(* Logix 5000 Routine export GOV_Plus_Program; software revision 20.01 *)

TYPE GOVPlus_Output :
STRUCT
   Target : DINT;
   Actuator_Control : INT;
   StatusControl : INT;
   Stop : BOOL;
   Reserved18 : BOOL;
   Reserved19 : BOOL;
   Reserved20 : BOOL;
   Reserved21 : BOOL;
   Reserved22 : BOOL;
   Reserved23 : BOOL;
   Reserved24 : BOOL;
   Reserved25 : BOOL;
   Reserved26 : BOOL;
   Reserved27 : BOOL;
   Reserved28 : BOOL;
   Reserved29 : BOOL;
   SW1_Failsafe : BOOL;
   SW1_Latching : BOOL;
   SW1_Enabled : BOOL;
   Spare : INT;
   Aux_Out : REAL;
   Float_Val : DINT;
   Float_Div : DINT;
END_STRUCT
END_TYPE

TYPE GOVPlus_ProgramData :
STRUCT
   GOV_ComCode : INT;
   GOV_ComCount : INT;
   GOV_Reconfigure : BOOL;
   Refresh_Stop_Data : BOOL;
   Refresh_ONS : BOOL;
   Stop_ONS : BOOL;
   Stop_Out_at_Stop : BOOL;
   Safety_Loop_at_Stop : BOOL;
   Actuator_Mode_Backup : BOOL;
   Current_Limit_Backup : BOOL;
   Reconfigure_Req : BOOL;
   Reconfigure_ONS : BOOL;
   Load_Defaults : BOOL;
   Limit_Low : REAL;
   Limit_High : REAL;
   Aux_Limit_Low : REAL;
   Aux_Limit_High : REAL;
   Stop_Data : GOV_Stop_Data;
   Gearteeth_Backup : INT;
   Start_Speed_Backup : DINT;
   Crank_Speed_Backup : DINT;
   Overspeed_Backup : DINT;
   Output_at_0_Percent_Backup : REAL;
   Output_at_100_Percent_Backup : REAL;
END_STRUCT
END_TYPE

TYPE GOVPlus_Input :
STRUCT
   Reserved1 : BOOL;
   Reserved2 : BOOL;
   V3_3Low : BOOL;
   V3_3High : BOOL;
   V5Low : BOOL;
   V5High : BOOL;
   V12_5Low : BOOL;
   V12_5High : BOOL;
   V24Low : BOOL;
   V24High : BOOL;
   AuxLoopLow : BOOL;
   AuxLoopHigh : BOOL;
   Reserved13 : BOOL;
   Reserved14 : BOOL;
   DemandLoopLow : BOOL;
   DemandLoopHigh : BOOL;
   CoolDownInputStatus : BOOL;
   StopInputStatus : BOOL;
   CurrentLoopOutputOpen : BOOL;
   SW1_Enabled_Echo : BOOL;
   SW1_Latching_Echo : BOOL;
   SW1_Failsafe_Echo : BOOL;
   Reserved23 : BOOL;
   Rotating : BOOL;
   AlarmOutActive : BOOL;
   StopOutClosed : BOOL;
   AuxOutputOutOfRange : BOOL;
   Target_Met : BOOL;
   Stop_Echo : BOOL;
   Reserved30 : BOOL;
   VoltOutActive : BOOL;
   V12_5SupplyFaulted : BOOL;
   Breaking : BOOL;
   WatchdogFailure : BOOL;
   FactoryCalEnabled : BOOL;
   WatchdogInhibited : BOOL;
   ActuatorEnabled : BOOL;
   Governing : BOOL;
   Timer1Active : BOOL;
   Timer2Active : BOOL;
   Timer3Active : BOOL;
   Purging : BOOL;
   Cooldown : BOOL;
   Max_Authority : BOOL;
   Demand_Active : BOOL;
   Target_Active : BOOL;
   Voltage_Driver_Output_On : BOOL;
   Reserved48 : BOOL;
   Aux_Output_Alarm : BOOL;
   Actuator_Output_Fault : BOOL;
   Overspeed : BOOL;
   Underspeed : BOOL;
   Stopped : BOOL;
   Reserved54 : BOOL;
   Reserved55 : BOOL;
   Reserved56 : BOOL;
   Reserved57 : BOOL;
   Reserved58 : BOOL;
   Reserved59 : BOOL;
   Reserved60 : BOOL;
   Reserved61 : BOOL;
   Reserved62 : BOOL;
   Reserved63 : BOOL;
   Reserved64 : BOOL;
   GovTime : REAL;
   Accelleration : REAL;
   RPM : DINT;
   RPMUnfiltered : REAL;
   DemandInput : REAL;
   AuxInput : REAL;
   CurrentOut : REAL;
   VoltageOut : REAL;
   Voltage_240 : REAL;
   Voltage_100 : REAL;
   Voltage_50 : REAL;
   Voltage_33 : REAL;
   Voltage_Output_Sense_Value : REAL;
   DemandTarget : DINT;
   ProcessorUsage : INT;
   GovState : INT;
   Speed_Target : REAL;
   Acceleration_Target : REAL;
   Acceleration_Error : REAL;
   RPM_Error : INT;
   Actuator_Position_Output : INT;
   ActuatorCounts : DINT;
   UpWindow : INT;
   DownWindow : INT;
   Float_Rsp : REAL;
   Comm_Status : INT;
   Spare_Echo : INT;
   Aux_Out_Echo : REAL;
END_STRUCT
END_TYPE

TYPE GOV_Stop_Data :
STRUCT
   Warmup_1 : BOOL;
   Warmup_2 : BOOL;
   Warmup_3 : BOOL;
   Cooldown : BOOL;
   Demand : BOOL;
   Purging : BOOL;
   Actuator_Offline : BOOL;
   Governing : BOOL;
   Braking : BOOL;
   Max_Authority : BOOL;
   Target_Met : BOOL;
   Underspeed : BOOL;
   Alarm : BOOL;
   V24Problem : BOOL;
   V12Problem : BOOL;
   PowerProblem : BOOL;
   Actuator_Output : INT;
   Target : DINT;
   RPM : DINT;
   Acceleration : INT;
   RPM_Error : INT;
   Acceleration_Target : INT;
   Acceleration_Error : INT;
   Actuator_Position : INT;
   Reserved : INT;
END_STRUCT
END_TYPE

VAR_GLOBAL   (* controller tags *)
   GOV_Input : GOVPlus_Input := (SW1_Enabled_Echo := 1, SW1_Latching_Echo := 1, SW1_Failsafe_Echo := 1, AlarmOutActive := 1, StopOutClosed := 1, Stop_Echo := 1, VoltOutActive := 1, WatchdogFailure := 1, Demand_Active := 1, Target_Active := 1, Underspeed := 1, DemandInput := 18.0, AuxInput := 4.959961, CurrentOut := 4.0, VoltageOut := 9.98999, Voltage_240 := 22.899902, Voltage_100 := 12.399902, Voltage_50 := 5.2999268, Voltage_33 := 3.1999512, Voltage_Output_Sense_Value := 9.899902, DemandTarget := 1801, ProcessorUsage := 34, UpWindow := 5, DownWindow := 5, Float_Rsp := 2.3999634, Aux_Out_Echo := 10.0);
   GOV_Stop_MSG : MESSAGE;
        MessageParameters(MessageType := CIP Generic, ConnectedFlag := 2, ConnectionPath := GOVPlus, ServiceCode := 16#0001, ObjectType := 16#006e, TargetObject := 1, DestinationTag := GOV_Program_Data.Stop_Data)
   GOVPlus_NFO : MESSAGE;
        MessageParameters(MessageType := Module Reconfigure, RequestedLength := 1, ConnectionPath := GOVPlus)
   GOV_Output : GOVPlus_Output := (Target := 1800, Actuator_Control := 15, Stop := 1, SW1_Failsafe := 1, SW1_Latching := 1, SW1_Enabled := 1, Aux_Out := 10.0, Float_Val := 240, Float_Div := 100);
   GOV_Program_Data : GOVPlus_ProgramData := (Actuator_Mode_Backup := 1, Limit_Low := 4.0, Limit_High := 20.0, Aux_Limit_High := 10.0, Stop_Data.Underspeed := 1, Stop_Data.Alarm := 1, Gearteeth_Backup := 60, Start_Speed_Backup := 150, Crank_Speed_Backup := 50, Overspeed_Backup := 2000, Output_at_0_Percent_Backup := 4.0, Output_at_100_Percent_Backup := 20.0);
END_VAR

PROGRAM DET_COM

ROUTINE GOV_Plus_Program   (* ladder *)
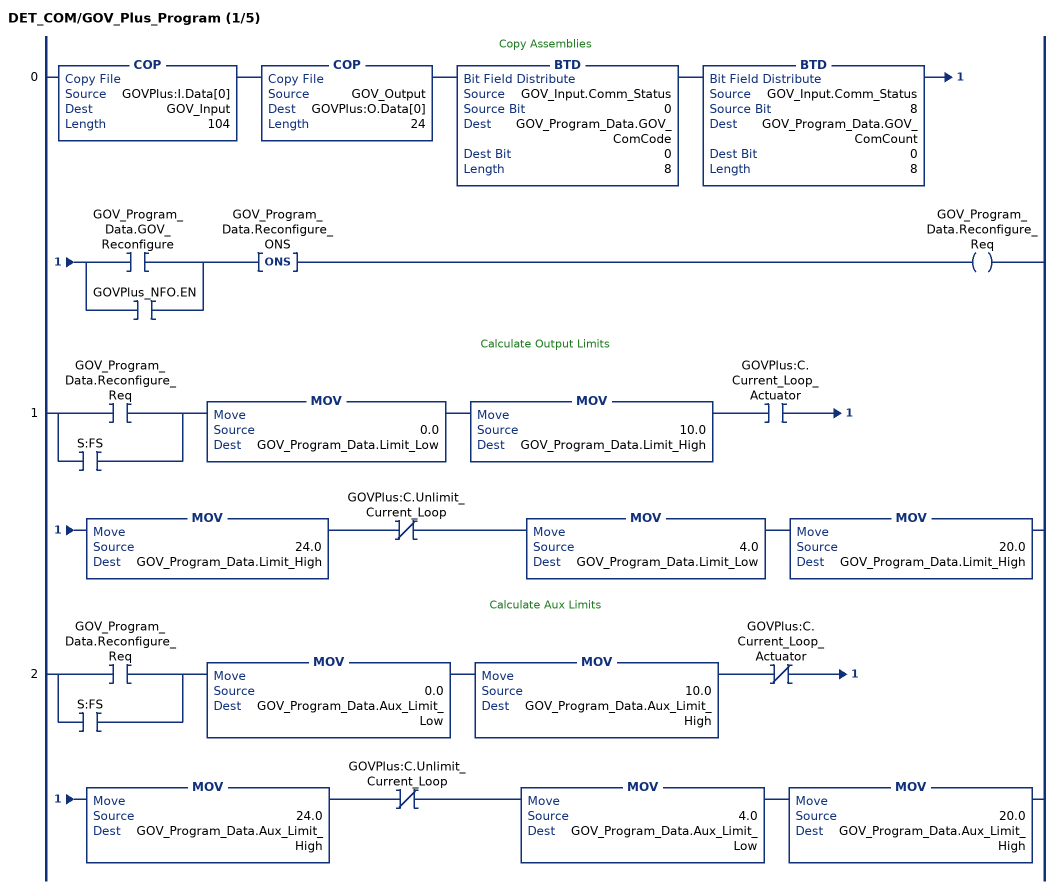
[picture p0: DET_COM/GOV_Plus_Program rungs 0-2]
   // Copy Assemblies
   0: COP(GOVPlus:I.Data[0],GOV_Input,104)COP(GOV_Output,GOVPlus:O.Data[0],24)BTD(GOV_Input.Comm_Status,0,GOV_Program_Data.GOV_ComCode,0,8)BTD(GOV_Input.Comm_Status,8,GOV_Program_Data.GOV_ComCount,0,8)[XIC(GOV_Program_Data.GOV_Reconfigure) ,XIC(GOVPlus_NFO.EN) ]ONS(GOV_Program_Data.Reconfigure_ONS)OTE(GOV_Program_Data.Reconfigure_Req);
   // Calculate Output Limits
   1: [XIC(GOV_Program_Data.Reconfigure_Req) ,XIC(S:FS) ]MOV(0.0,GOV_Program_Data.Limit_Low)MOV(10.0,GOV_Program_Data.Limit_High)XIC(GOVPlus:C.Current_Loop_Actuator)MOV(24.0,GOV_Program_Data.Limit_High)XIO(GOVPlus:C.Unlimit_Current_Loop)MOV(4.0,GOV_Program_Data.Limit_Low)MOV(20.0,GOV_Program_Data.Limit_High);
   // Calculate Aux Limits
   2: [XIC(GOV_Program_Data.Reconfigure_Req) ,XIC(S:FS) ]MOV(0.0,GOV_Program_Data.Aux_Limit_Low)MOV(10.0,GOV_Program_Data.Aux_Limit_High)XIO(GOVPlus:C.Current_Loop_Actuator)MOV(24.0,GOV_Program_Data.Aux_Limit_High)XIO(GOVPlus:C.Unlimit_Current_Loop)MOV(4.0,GOV_Program_Data.Aux_Limit_Low)MOV(20.0,GOV_Program_Data.Aux_Limit_High);
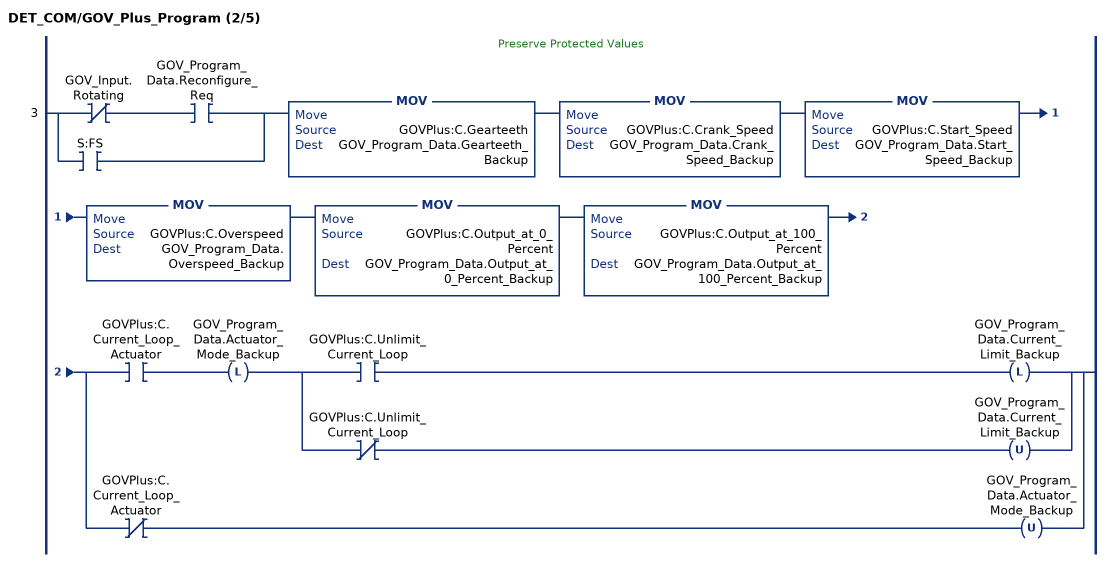
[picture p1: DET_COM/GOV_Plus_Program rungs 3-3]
   // Preserve Protected Values
   3: [XIO(GOV_Input.Rotating) XIC(GOV_Program_Data.Reconfigure_Req) ,XIC(S:FS) ]MOV(GOVPlus:C.Gearteeth,GOV_Program_Data.Gearteeth_Backup)MOV(GOVPlus:C.Crank_Speed,GOV_Program_Data.Crank_Speed_Backup)MOV(GOVPlus:C.Start_Speed,GOV_Program_Data.Start_Speed_Backup)MOV(GOVPlus:C.Overspeed,GOV_Program_Data.Overspeed_Backup)MOV(GOVPlus:C.Output_at_0_Percent,GOV_Program_Data.Output_at_0_Percent_Backup)MOV(GOVPlus:C.Output_at_100_Percent,GOV_Program_Data.Output_at_100_Percent_Backup)[XIC(GOVPlus:C.Current_Loop_Actuator) OTL(GOV_Program_Data.Actuator_Mode_Backup) [XIC(GOVPlus:C.Unlimit_Current_Loop) OTL(GOV_Program_Data.Current_Limit_Backup) ,XIO(GOVPlus:C.Unlimit_Current_Loop) OTU(GOV_Program_Data.Current_Limit_Backup) ] ,XIO(GOVPlus:C.Current_Loop_Actuator) OTU(GOV_Program_Data.Actuator_Mode_Backup) ];
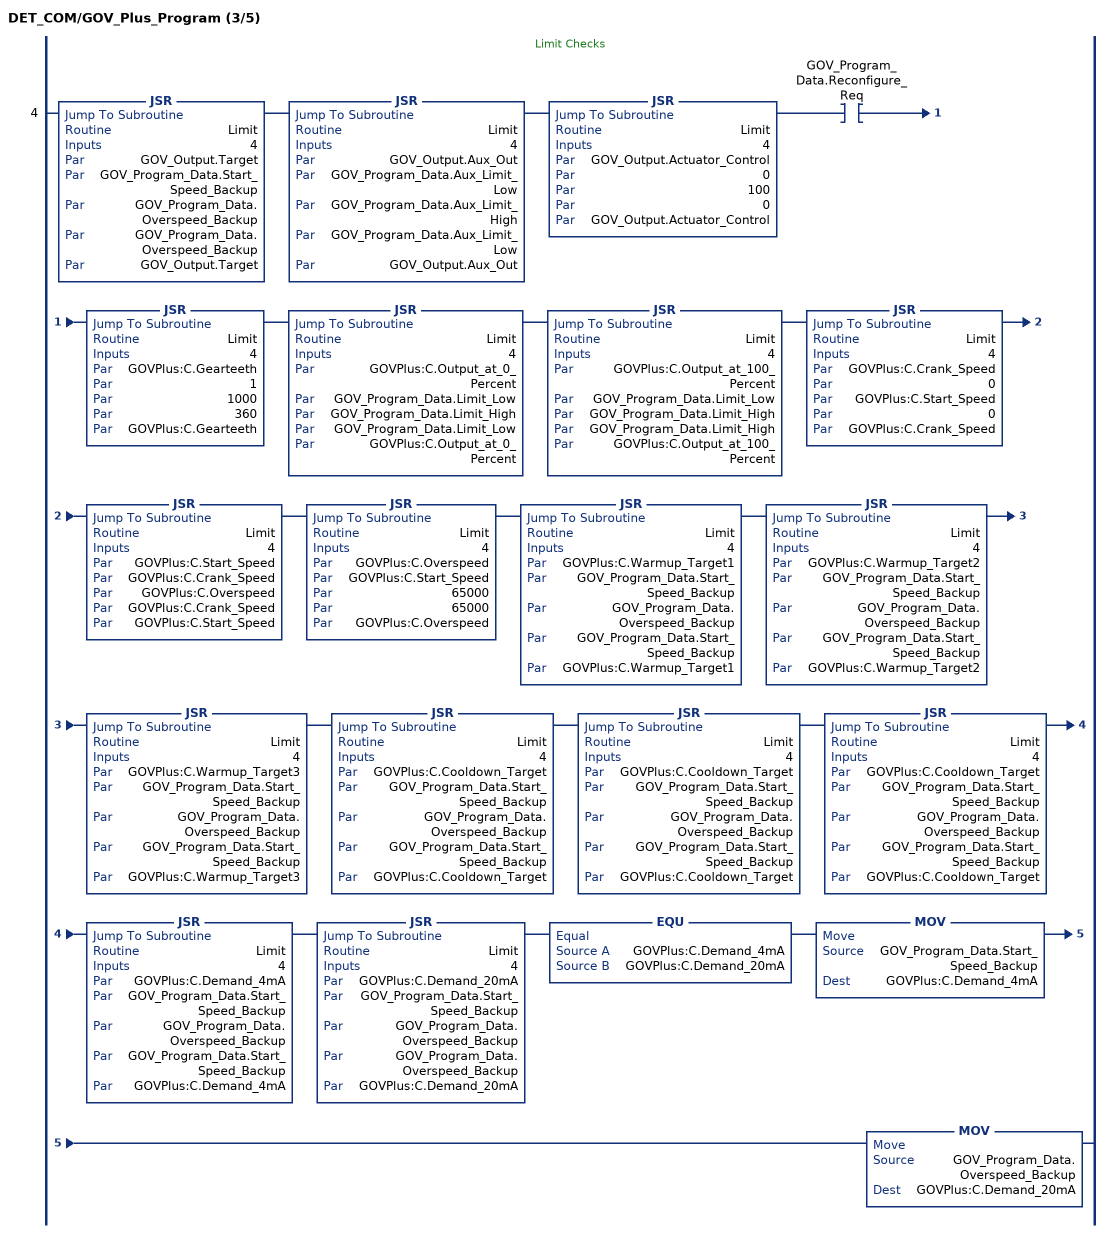
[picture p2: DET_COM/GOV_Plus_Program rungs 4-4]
   // Limit Checks
   4: JSR(Limit,4,GOV_Output.Target,GOV_Program_Data.Start_Speed_Backup,GOV_Program_Data.Overspeed_Backup,GOV_Program_Data.Overspeed_Backup,GOV_Output.Target)JSR(Limit,4,GOV_Output.Aux_Out,GOV_Program_Data.Aux_Limit_Low,GOV_Program_Data.Aux_Limit_High,GOV_Program_Data.Aux_Limit_Low,GOV_Output.Aux_Out)JSR(Limit,4,GOV_Output.Actuator_Control,0,100,0,GOV_Output.Actuator_Control)XIC(GOV_Program_Data.Reconfigure_Req)JSR(Limit,4,GOVPlus:C.Gearteeth,1,1000,360,GOVPlus:C.Gearteeth)JSR(Limit,4,GOVPlus:C.Output_at_0_Percent,GOV_Program_Data.Limit_Low,GOV_Program_Data.Limit_High,GOV_Program_Data.Limit_Low,GOVPlus:C.Output_at_0_Percent)JSR(Limit,4,GOVPlus:C.Output_at_100_Percent,GOV_Program_Data.Limit_Low,GOV_Program_Data.Limit_High,GOV_Program_Data.Limit_High,GOVPlus:C.Output_at_100_Percent)JSR(Limit,4,GOVPlus:C.Crank_Speed,0,GOVPlus:C.Start_Speed,0,GOVPlus:C.Crank_Speed)JSR(Limit,4,GOVPlus:C.Start_Speed,GOVPlus:C.Crank_Speed,GOVPlus:C.Overspeed,GOVPlus:C.Crank_Speed,GOVPlus:C.Start_Speed)JSR(Limit,4,GOVPlus:C.Overspeed,GOVPlus:C.Start_Speed,65000,65000,GOVPlus:C.Overspeed)JSR(Limit,4,GOVPlus:C.Warmup_Target1,GOV_Program_Data.Start_Speed_Backup,GOV_Program_Data.Overspeed_Backup,GOV_Program_Data.Start_Speed_Backup,GOVPlus:C.Warmup_Target1)JSR(Limit,4,GOVPlus:C.Warmup_Target2,GOV_Program_Data.Start_Speed_Backup,GOV_Program_Data.Overspeed_Backup,GOV_Program_Data.Start_Speed_Backup,GOVPlus:C.Warmup_Target2)JSR(Limit,4,GOVPlus:C.Warmup_Target3,GOV_Program_Data.Start_Speed_Backup,GOV_Program_Data.Overspeed_Backup,GOV_Program_Data.Start_Speed_Backup,GOVPlus:C.Warmup_Target3)JSR(Limit,4,GOVPlus:C.Cooldown_Target,GOV_Program_Data.Start_Speed_Backup,GOV_Program_Data.Overspeed_Backup,GOV_Program_Data.Start_Speed_Backup,GOVPlus:C.Cooldown_Target)JSR(Limit,4,GOVPlus:C.Cooldown_Target,GOV_Program_Data.Start_Speed_Backup,GOV_Program_Data.Overspeed_Backup,GOV_Program_Data.Start_Speed_Backup,GOVPlus:C.Cooldown_Target)JSR(Limit,4,GOVPlus:C.Cooldown_Target,GOV_Program_Data.Start_Speed_Backup,GOV_Program_Data.Overspeed_Backup,GOV_Program_Data.Start_Speed_Backup,GOVPlus:C.Cooldown_Target)JSR(Limit,4,GOVPlus:C.Demand_4mA,GOV_Program_Data.Start_Speed_Backup,GOV_Program_Data.Overspeed_Backup,GOV_Program_Data.Start_Speed_Backup,GOVPlus:C.Demand_4mA)JSR(Limit,4,GOVPlus:C.Demand_20mA,GOV_Program_Data.Start_Speed_Backup,GOV_Program_Data.Overspeed_Backup,GOV_Program_Data.Overspeed_Backup,GOVPlus:C.Demand_20mA)EQU(GOVPlus:C.Demand_4mA,GOVPlus:C.Demand_20mA)MOV(GOV_Program_Data.Start_Speed_Backup,GOVPlus:C.Demand_4mA)MOV(GOV_Program_Data.Overspeed_Backup,GOVPlus:C.Demand_20mA);
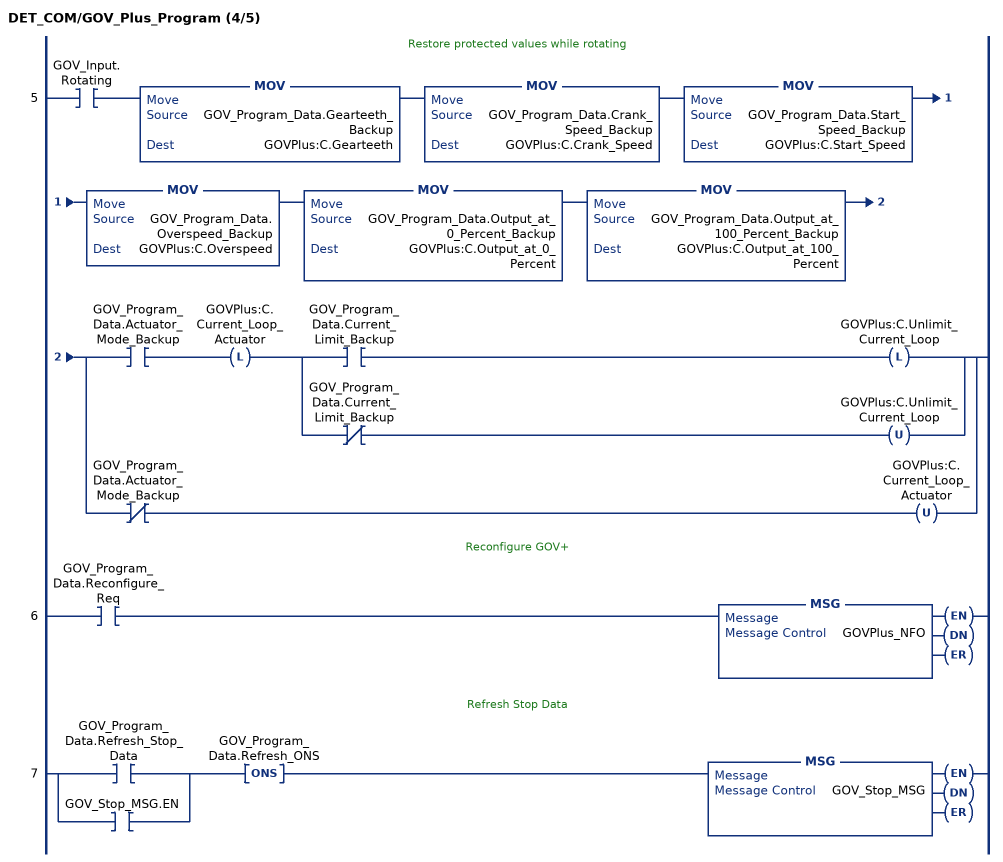
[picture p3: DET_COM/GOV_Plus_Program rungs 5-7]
   // Restore protected values while rotating
   5: XIC(GOV_Input.Rotating)MOV(GOV_Program_Data.Gearteeth_Backup,GOVPlus:C.Gearteeth)MOV(GOV_Program_Data.Crank_Speed_Backup,GOVPlus:C.Crank_Speed)MOV(GOV_Program_Data.Start_Speed_Backup,GOVPlus:C.Start_Speed)MOV(GOV_Program_Data.Overspeed_Backup,GOVPlus:C.Overspeed)MOV(GOV_Program_Data.Output_at_0_Percent_Backup,GOVPlus:C.Output_at_0_Percent)MOV(GOV_Program_Data.Output_at_100_Percent_Backup,GOVPlus:C.Output_at_100_Percent)[XIC(GOV_Program_Data.Actuator_Mode_Backup) OTL(GOVPlus:C.Current_Loop_Actuator) [XIC(GOV_Program_Data.Current_Limit_Backup) OTL(GOVPlus:C.Unlimit_Current_Loop) ,XIO(GOV_Program_Data.Current_Limit_Backup) OTU(GOVPlus:C.Unlimit_Current_Loop) ] ,XIO(GOV_Program_Data.Actuator_Mode_Backup) OTU(GOVPlus:C.Current_Loop_Actuator) ];
   // Reconfigure GOV+
   6: XIC(GOV_Program_Data.Reconfigure_Req)MSG(GOVPlus_NFO);
   // Refresh Stop Data
   7: [XIC(GOV_Program_Data.Refresh_Stop_Data) ,XIC(GOV_Stop_MSG.EN) ]ONS(GOV_Program_Data.Refresh_ONS)MSG(GOV_Stop_MSG);
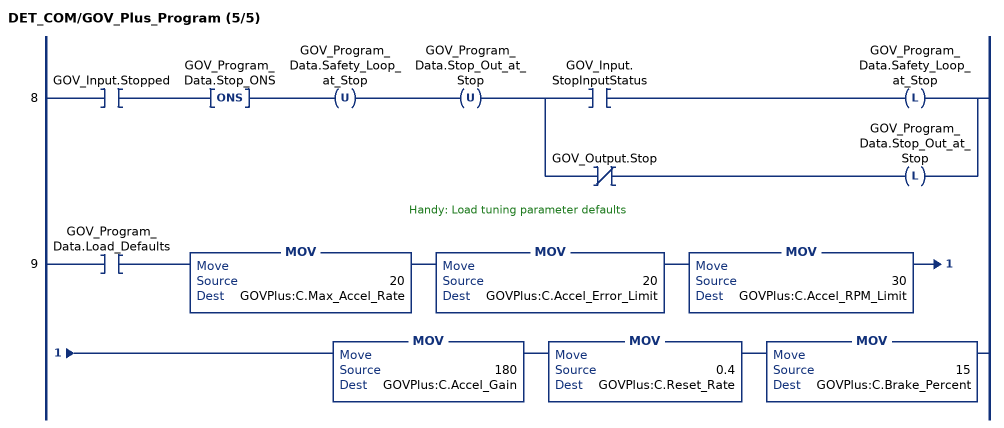
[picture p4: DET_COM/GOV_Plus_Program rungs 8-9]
   8: XIC(GOV_Input.Stopped)ONS(GOV_Program_Data.Stop_ONS)OTU(GOV_Program_Data.Safety_Loop_at_Stop)OTU(GOV_Program_Data.Stop_Out_at_Stop)[XIC(GOV_Input.StopInputStatus) OTL(GOV_Program_Data.Safety_Loop_at_Stop) ,XIO(GOV_Output.Stop) OTL(GOV_Program_Data.Stop_Out_at_Stop) ];
   // Handy: Load tuning parameter defaults
   9: XIC(GOV_Program_Data.Load_Defaults)MOV(20,GOVPlus:C.Max_Accel_Rate)MOV(20,GOVPlus:C.Accel_Error_Limit)MOV(30,GOVPlus:C.Accel_RPM_Limit)MOV(180,GOVPlus:C.Accel_Gain)MOV(0.4,GOVPlus:C.Reset_Rate)MOV(15,GOVPlus:C.Brake_Percent);
END_ROUTINE
END_PROGRAM
